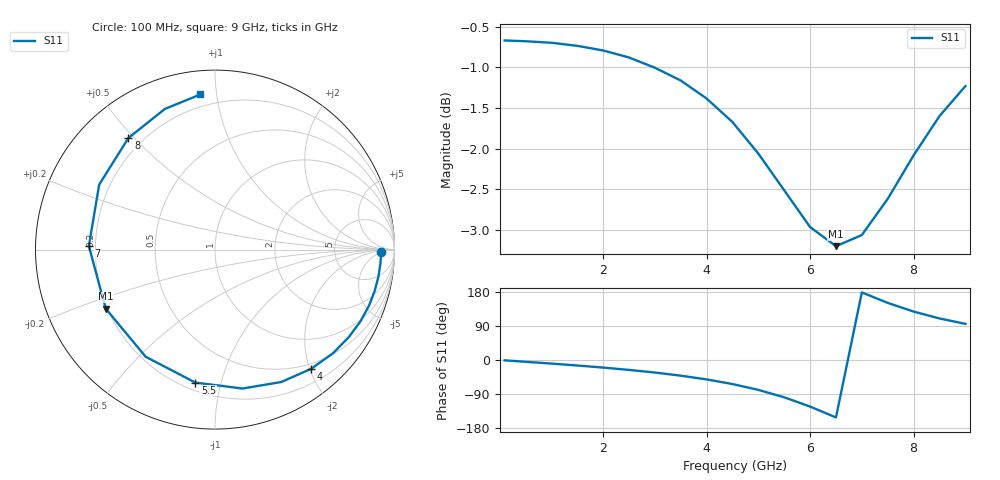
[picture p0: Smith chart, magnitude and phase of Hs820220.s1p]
!HSMS-8101 and HSMS-8202 Schottky diodes
!S-parameters at 20 microamp external bias.  Last updated 6/7/94
# ghz s ma r 50
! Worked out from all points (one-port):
!   19 points, 100 MHz to 9 GHz, reference 50 ohm
!   lowest |S11| = -3.2 dB at 6.5 GHz (marker M1), VSWR 5.49, Z = 9.66 - j12.2 ohm
!   |S11| at or under -10 dB: nowhere
!   S11 on the Smith chart (normalised r, x): 100 MHz: 25, -5; 4 GHz: 0.41, -2.02; 5.5 GHz: 0.25, -0.83; 7 GHz: 0.17, +0.01; 8 GHz: 0.15, +0.48; 9 GHz: 0.13, +0.90
0.1  0.926 -0.9
0.5  0.925 -4.7
1  0.923 -9.4
1.5  0.919 -14.5
2  0.913 -20.0
2.5  0.904 -26.1
3  0.891 -33.1
3.5  0.875 -41.3
4  0.853 -51.2
4.5  0.825 -63.4
5  0.789 -78.8
5.5  0.749 -98.4
6  0.711 -122.9
6.5  0.692 -151.6
7  0.703 178.4
7.5  0.74 150.7
8  0.787 127.8
8.5  0.832 109.6
9  0.868 95.4
